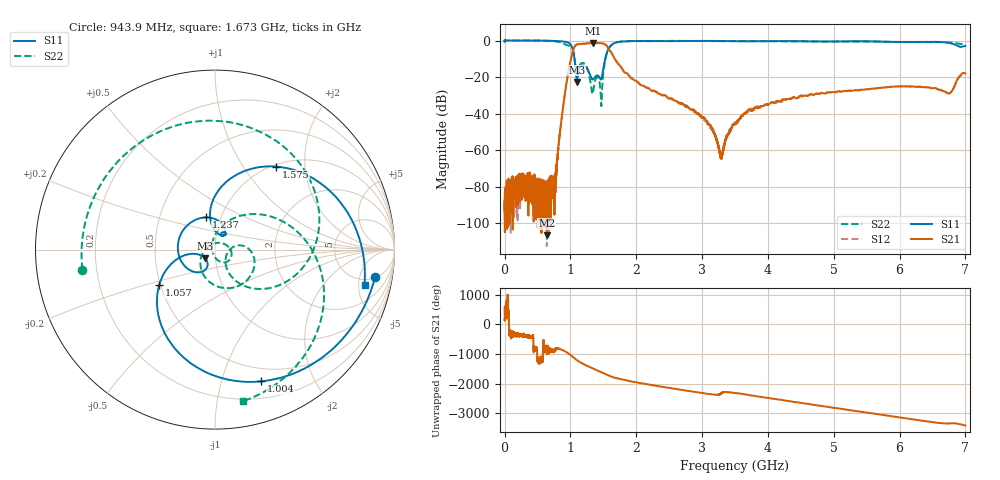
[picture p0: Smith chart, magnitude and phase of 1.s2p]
!Keysight Technologies,N5232A,MY52221221,A.10.65.11
!Date: Thursday, February 23, 2023 13:27:19
!Correction: S11(Full 2 Port(1,4))
!S41(Full 2 Port(1,4))
!S14(Full 2 Port(1,4))
!S44(Full 2 Port(1,4))
!S2P File: Measurements: S11, S41, S14, S44:
# Hz S  RI  R 50
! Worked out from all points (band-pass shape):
!   16001 points, 300 kHz to 7 GHz, reference 50 ohm
!   highest |S21| = -1.38 dB at 1.344 GHz (marker M1); lowest = -106.4 dB at 641.6 MHz (marker M2)
!   |S21| within 3 dB of the highest: 1.049 GHz to 1.578 GHz (528.9 MHz wide, 40.3 % of centre)
!   lowest |S11| = -22.7 dB at 1.098 GHz (marker M3), VSWR 1.16, Z = 44.7 - j4.43 ohm
!   |S11| at or under -10 dB: 1.062 GHz to 1.528 GHz (466 MHz wide, 36 % of centre)
!   |S22| runs from -35.9 to 0.0 dB; largest |S21 - S12| = 0.018
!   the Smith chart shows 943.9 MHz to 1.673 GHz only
!   S11 on the Smith chart (normalised r, x): 943.9 MHz: 5, -9; 1.004 GHz: 0.36, -1.35; 1.057 GHz: 0.49, -0.22; 1.237 GHz: 0.85, +0.32; 1.575 GHz: 1.03, +1.43; 1.673 GHz: 3.95, -5.90
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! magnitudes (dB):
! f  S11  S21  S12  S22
! 300 kHz  0.0  -87.6  -82.8  0.0
! 641.6 MHz  -0.1  -106.4  -91.8  -0.2
! 766.3 MHz  -0.3  -76.1  -81.1  -0.5
! 943.9 MHz  -0.9  -22.4  -22.4  -2.5
! 1.004 GHz  -2.2  -10.7  -10.7  -3.1
! 1.057 GHz  -8.7  -3.7  -3.8  -8.4
! 1.098 GHz  -22.7  -2.2  -2.2  -23.0
! 1.167 GHz  -13.8  -1.8  -2.0  -12.4
! 1.237 GHz  -14.6  -1.7  -1.7  -13.7
! 1.344 GHz  -21.3  -1.4  -1.3  -27.7
! 1.404 GHz  -19.1  -1.4  -1.4  -20.0
! 1.472 GHz  -20.8  -1.5  -1.5  -35.3
! 1.575 GHz  -4.8  -4.1  -4.2  -5.0
! 1.673 GHz  -1.3  -10.0  -9.8  -1.3
! 2.334 GHz  -0.3  -29.0  -28.4  -0.3
! 3.032 GHz  -0.2  -42.2  -43.2  -0.4
! 3.288 GHz  -0.3  -64.0  -64.3  -0.4
! 3.5 GHz  -0.4  -45.7  -44.8  -0.3
! 4.667 GHz  -0.5  -29.5  -29.1  -0.5
! 5.834 GHz  -0.7  -25.4  -25.4  -0.7
! 6.751 GHz  -1.3  -29.1  -28.8  -1.0
! 7 GHz  -3.0  -18.0  -18.2  -2.3
